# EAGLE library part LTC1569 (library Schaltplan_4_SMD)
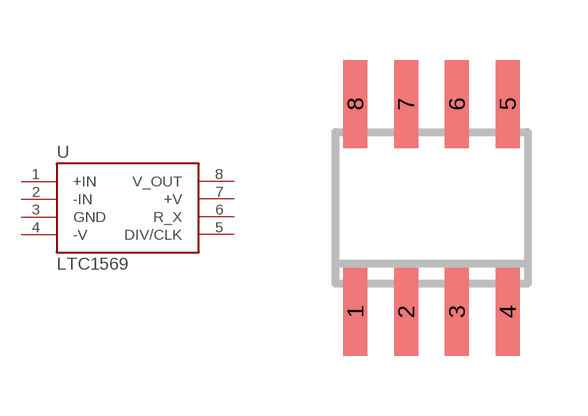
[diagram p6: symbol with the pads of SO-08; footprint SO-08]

Designator prefix -

## LTC1569  [SO-08]
1  +IN
2  -IN
3  GND
4  -V
5  DIV/CLK
6  R_X
7  +V
8  V_OUT

## Footprint SO-08 (pad centres in mm)
Small Outline Narrow Plastic Gull Wing 150-mil body, package type SN
smd 0.6 x 2.2: 1 -1.905,-2.6; 2 -0.635,-2.6; 3 0.635,-2.6; 4 1.905,-2.6; 5 1.905,2.6; 6 0.635,2.6; 7 -0.635,2.6; 8 -1.905,2.6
